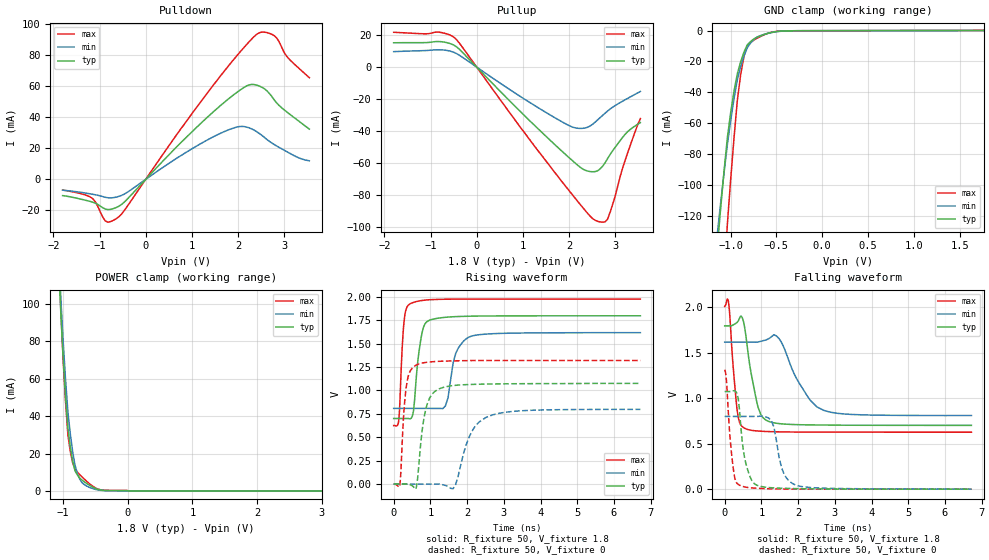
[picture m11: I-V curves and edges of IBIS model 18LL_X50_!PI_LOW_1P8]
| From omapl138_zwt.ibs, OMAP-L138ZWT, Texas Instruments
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|   Model Cell 18LL_X50_!PI_LOW_1P8
|BC1833DV40CTPBFZ_!PI_LOW_1P8
[Model]   18LL_X50_!PI_LOW_1P8
Model_type   I/O
Polarity   Non-Inverting
Enable   Active-Low
Vinl =  0.63
Vinh =  1.17
Cref =  15pF
Rref =  100.00M
Vref =  0V
Vmeas =  0.9
C_comp   2.232809p   2.073051p   2.295852p
[Model Spec]
Vinl   0.63   0.567   0.693
Vinh   1.17   1.053   1.287
[Temperature Range]   25   125   -40
[Voltage Range]   1.8   1.62   1.98
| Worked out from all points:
|   slope of the pulldown table from 0 to 0.27 V, typ, clamps not added: 31.4 ohm
|   slope of the pullup table from 0 to 0.27 V, typ, clamps not added: 33.4 ohm
|   GND clamp passes 1 mA (typ) near -0.54 V on its own axis
|   POWER clamp passes 1 mA (typ) near -0.48 V on its own axis
|   rising waveform, R_fixture 50, V_fixture 1.8: 20-80 % time 180ps typ, 267ps min, 104ps max; typ from 0.7 V to 1.8 V
|   rising waveform, R_fixture 50, V_fixture 0: 20-80 % time 232ps typ, 465ps min, 139ps max; typ from 0 V to 1.07 V
|   falling waveform, R_fixture 50, V_fixture 1.8: 20-80 % time 285ps typ, 637ps min, 162ps max; typ from 1.8 V to 0.702 V
|   falling waveform, R_fixture 50, V_fixture 0: 20-80 % time 220ps typ, 263ps min, 153ps max; typ from 1.07 V to 0 V
[POWER_clamp]
|   voltage   I(typ)   I(min)   I(max)
-1.8V     842.4mA    869.3mA    912.9mA
-1.073V   123.7mA    130.9mA    129.1mA
-1.036V   94.83mA    102.9mA    96.56mA
-1V       70.85mA    79.7mA     69.66mA
-963.6mV  50.44mA    59.51mA    47.46mA
-927.3mV  33.63mA    42.34mA    29.99mA
-890.9mV  23.71mA    30.8mA     21.26mA
-818.2mV  10.87mA    13.88mA    11.68mA
-781.8mV  8.623mA    9.578mA    10.15mA
-636.4mV  3.988mA    2.612mA    5.172mA
-345.5mV  234.4uA    145uA      345.5uA
3.6V      0A         0A         0A
[Pulldown]
|   voltage   I(typ)   I(min)   I(max)
-1.8V     -10.49mA   -6.992mA   -6.878mA
-1.145V   -14.77mA   -9.642mA   -12.54mA
-872.7mV  -19.17mA   -11.58mA   -26.88mA
-600mV    -17.64mA   -11.15mA   -24.61mA
1.636V    48.04mA    29.95mA    67.37mA
2.073V    58.21mA    34.18mA    83.2mA
2.291V    61.28mA    32.65mA    90.41mA
2.455V    60.33mA    29.78mA    94.55mA
2.618V    57.37mA    25.94mA    94.82mA
2.782V    51.43mA    22.55mA    92.84mA
3.055V    43.59mA    17.92mA    79.47mA
3.545V    32.43mA    11.97mA    65.61mA
[Pullup]
|   voltage   I(typ)   I(min)   I(max)
-1.8V     15.27mA    9.71mA     21.85mA
-818.2mV  16.05mA    10.88mA    21.94mA
-490.9mV  13.72mA    9.222mA    18.66mA
1.036V    -30.46mA   -20.11mA   -41.15mA
2.018V    -57.22mA   -36.91mA   -78.08mA
2.345V    -64.63mA   -38.19mA   -89.73mA
2.618V    -65.01mA   -33.11mA   -96.69mA
2.782V    -59.96mA   -28.87mA   -97.07mA
2.836V    -57.31mA   -27.51mA   -95.25mA
3V        -50.25mA   -24.09mA   -80.86mA
3.218V    -42.03mA   -20.43mA   -58.16mA
3.545V    -34.78mA   -15.26mA   -32.29mA
[GND_clamp]
|   voltage   I(typ)   I(min)   I(max)
-1.8V     -697.8mA   -553.2mA   -1.259A
-1.145V   -140.7mA   -131.7mA   -248.3mA
-1.109V   -115.1mA   -111.6mA   -203.3mA
-1.036V   -69.61mA   -74.07mA   -125.9mA
-963.6mV  -39.29mA   -44.18mA   -69.68mA
-927.3mV  -27.97mA   -31.86mA   -45.36mA
-890.9mV  -20.15mA   -23.34mA   -28.44mA
-854.5mV  -13.89mA   -16.39mA   -16.54mA
-818.2mV  -9.198mA   -11.01mA   -9.648mA
-709.1mV  -4.172mA   -4.037mA   -4.792mA
-418.2mV  -167.1uA   -231.6uA   -161.9uA
1.764V    148.6uA    81.79uA    236.4uA
[Ramp]
| variable   typ   min   max
dV/dt_f  0.7217987/0.2986319n   0.53461/0.6646511n  0.8809398/0.1679611n
dV/dt_r  0.6786641/0.2305213n  0.5125735/0.4703193n  0.8110502/0.1380863n
R_load = 50
[Rising Waveform]
R_fixture = 50
V_fixture = 1.8
V_fixture_min = 1.62
V_fixture_max = 1.98
|   time   V(typ)   V(min)   V(max)
0s        700.4mV    808.1mV    624.7mV
140ps     700.4mV    808.1mV    682.9mV
280ps     700mV      808.1mV    1.723V
450ps     695.7mV    808.1mV    1.925V
770ps     1.61V      808.1mV    1.96V
980ps     1.75V      808mV      1.968V
1.41ns    1.781V     835.4mV    1.974V
1.69ns    1.788V     1.396V     1.975V
2.12ns    1.793V     1.58V      1.975V
6.72ns    1.797V     1.617V     1.976V
[Rising Waveform]
R_fixture = 50
V_fixture = 0
V_fixture_min = 0
V_fixture_max = 0
|   time   V(typ)   V(min)   V(max)
0s        -1.103uV   -197.3nV   -628.1uV
170ps     -2.458uV   3.374uV    -8.72mV
340ps     -493.6uV   428.8nV    1.027V
620ps     -30.77mV   434.4nV    1.271V
880ps     806.8mV    12.95uV    1.299V
1.26ns    1.02V      295.8uV    1.311V
1.62ns    1.052V     -49.11mV   1.315V
2.12ns    1.064V     555mV      1.319V
2.7ns     1.069V     739.4mV    1.319V
6.72ns    1.075V     797.5mV    1.319V
[Falling Waveform]
R_fixture = 50
V_fixture = 1.8
V_fixture_min = 1.62
V_fixture_max = 1.98
|   time   V(typ)   V(min)   V(max)
0s        1.797V     1.618V     2.012V
100ps     1.797V     1.618V     2.07V
340ps     1.837V     1.618V     866.3mV
540ps     1.789V     1.618V     670.9mV
910ps     901mV      1.62V      640.1mV
1.19ns    747mV      1.654V     634mV
1.48ns    721.8mV    1.658V     631.1mV
2.05ns    709.3mV    1.154V     628.7mV
2.7ns     705.9mV    867mV      627.9mV
6.72ns    702.4mV    810.6mV    627.3mV
[Falling Waveform]
R_fixture = 50
V_fixture = 0
V_fixture_min = 0
V_fixture_max = 0
|   time   V(typ)   V(min)   V(max)
0s        1.075V     800.7mV    1.315V
50ps      1.075V     800.7mV    1.183V
230ps     1.083V     800.7mV    239.3mV
400ps     885.8mV    800.7mV    44.92mV
570ps     294.3mV    800.7mV    22.46mV
910ps     38.56mV    800.8mV    9.815mV
1.26ns    16.05mV    760.1mV    3.968mV
1.62ns    9.431mV    163.8mV    1.465mV
1.97ns    5.88mV     40.07mV    551.7uV
6.72ns    58.95uV    1.373mV    5.977uV
